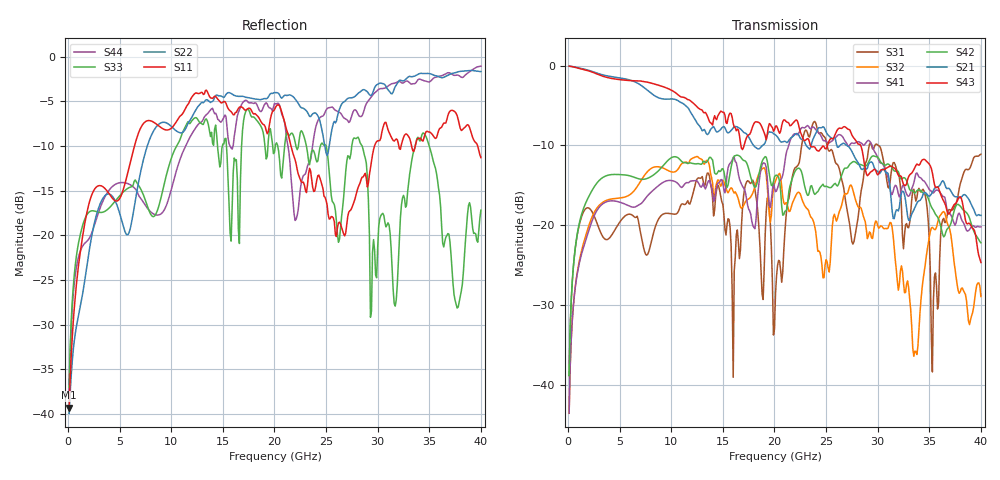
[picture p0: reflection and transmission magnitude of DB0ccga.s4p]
! ADC12DJ3200QML-SP
! 196-pin NWE package
! CCGA Ceramic Package with columns (ceramic column grid array)
! Texas Instruments 4/21/2021
! Single-ended  S-parameters
! PORT#  PORT_NAME  NET_NAME
! PORT1:  DAxN.DIEBUMP DAxN
! PORT2:  DAxN.BGA  DAxN
! PORT3:  DAxP.DIEBUMP DAxP
! PORT4:  DAxP.BGA  DAxP
! Touchstone Ver. 1.0
! Number of ports is 4
# Hz	S	MA	R	50.000000
! SCATTERING PARAMETERS  :
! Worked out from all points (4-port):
!   400 points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, 100 MHz to 40 GHz, reference 50 ohm
!   strongest paths, dB at 100 MHz, 10.1 GHz, 20.1 GHz, 30.1 GHz, 40 GHz:
!     S43: -0.1, -3.1, -7.6, -13.5, -24.7
!     S21: -0.1, -4.2, -8.7, -13.5, -18.8
!     S42: -38.8, -11.5, -13.7, -11.6, -22.2
!     S41: -43.5, -14.4, -15.8, -11.9, -20.2
!     S32: -43.5, -13.3, -14.5, -20.4, -28.9
!     S31: -38.8, -18.6, -28.6, -10.0, -11.1
!   lowest |S11| = -39.3 dB at 100 MHz (marker M1), VSWR 1.02, Z = 51 + j0.513 ohm
!   |S11| at or under -10 dB: start of sweep to 6.434 GHz; 21.6 GHz to 29.7 GHz (8.099 GHz wide, 31.6 % of centre); 33.28 GHz to 33.64 GHz (356.6 MHz wide, 1.07 % of centre)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
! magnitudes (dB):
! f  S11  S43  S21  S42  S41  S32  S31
! 100 MHz  -39.3  -0.1  -0.1  -38.8  -43.5  -43.5  -38.8
! 8.3 GHz  -7.3  -2.3  -3.7  -13.7  -15.5  -12.7  -20.8
! 16 GHz  -6.5  -7.3  -7.8  -11.6  -11.5  -15.7  -39.0
! 17.3 GHz  -5.9  -9.0  -8.6  -12.2  -16.8  -16.8  -14.6
! 29.9 GHz  -9.5  -13.5  -13.2  -11.4  -11.2  -19.5  -9.8
! 35.3 GHz  -8.7  -13.4  -15.9  -17.9  -15.9  -20.3  -38.4
! 40 GHz  -11.3  -24.7  -18.8  -22.2  -20.2  -28.9  -11.1
